VAR_GLOBAL
	ipCreator: I_AcsiCodeCreatorClass := GVL_AcsiVars.Creator.SetCodeRev(codeRev:=3).SetGuiVer(major:=1, minor:=1, build:=94, revision:=4);
	fbIED: FB_IED_IED;
	{warning 'Please configure your server IP-address in the initialization code of the client function block below:'}
	fbIEDClient: FB_IEDClient := (fbConnection:=(ipIED:=fbIED, settings:=(sRemoteHost:='127.0.0.1')));
END_VAR
